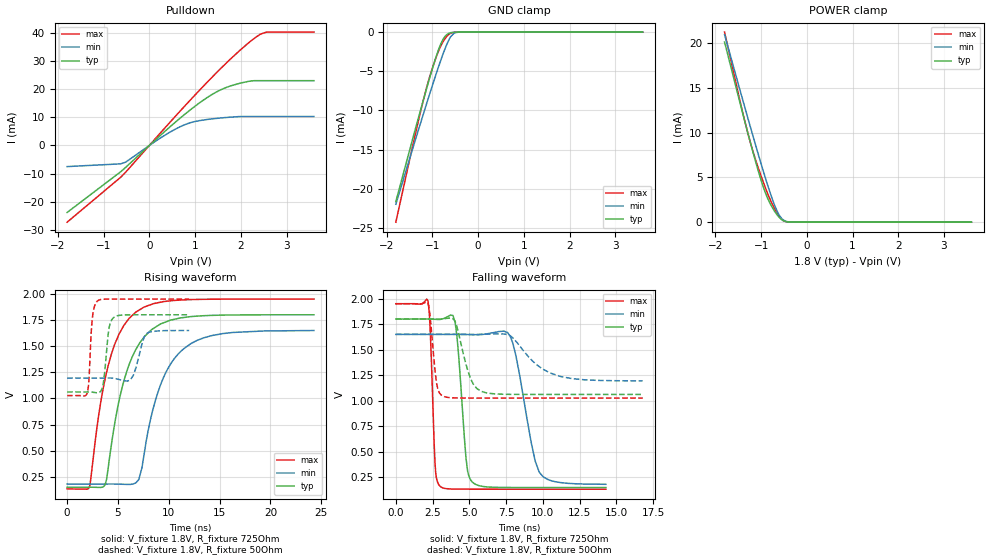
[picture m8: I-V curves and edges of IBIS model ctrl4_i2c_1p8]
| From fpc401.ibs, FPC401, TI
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|   ctrl4_i2c_1p8 Model
[Model]   ctrl4_i2c_1p8
Model_type   I/O_open_drain
Polarity   Non-Inverting
Vinl = 0.8
Vinh = 2
Vmeas = 0.9
Vref = 1.8
Cref = 50pF
Rref = 725
|   typ   min   max
|   (nom PVT)   (fast PVT)   (slow PVT)
C_comp   1.301e-14   1.196e-14   2.100e-14
| Where nom  PVT is Nominal Process, 1.8V, 27C
|   Fast PVT is Strong Process,  1.95V, -40C
|   Slow PVT is Weak Process,   1.65V, 125C
[Voltage Range]   1.8   1.65   1.95
|Junction Temperature
[Temperature Range]   27   125   -40
[Pullup Reference]   1.8   1.65   1.95
[Pulldown Reference]   0   0   0
[Power Clamp Reference]   1.8   1.65   1.95
[GND Clamp Reference]   0   0   0
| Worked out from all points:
|   slope of the pulldown table from 0 to 0.27 V, typ, clamps not added: 67.3 ohm
|   GND clamp passes 1 mA (typ) near -0.77 V on its own axis
|   POWER clamp passes 1 mA (typ) near -0.68 V on its own axis
|   falling waveform, V_fixture 1.8V, R_fixture 725Ohm: 20-80 % time 494ps typ, 1.1ns min, 265ps max; typ from 1.8 V to 0.152 V
|   rising waveform, V_fixture 1.8V, R_fixture 725Ohm: 20-80 % time 2.53ns typ, 2.78ns min, 2.33ns max; typ from 0.152 V to 1.8 V
|   falling waveform, V_fixture 1.8V, R_fixture 50Ohm: 20-80 % time 829ps typ, 2.01ns min, 364ps max; typ from 1.8 V to 1.06 V
|   rising waveform, V_fixture 1.8V, R_fixture 50Ohm: 20-80 % time 452ps typ, 746ps min, 317ps max; typ from 1.06 V to 1.8 V
[Pulldown]
|   Voltage   I(typ)   I(min)   I(max)
-1.8V     -23.87mA   -7.52mA    -27.33mA
-628mV    -9.35mA    -6.539mA   -11.32mA
-519.6mV  -7.811mA   -5.942mA   -9.523mA
251mV     3.762mA    2.768mA    4.649mA
682.2mV   9.87mA     6.746mA    12.43mA
1.012V    14.15mA    8.585mA    18.22mA
1.44V     18.83mA    9.603mA    25.46mA
1.649V    20.46mA    9.924mA    28.84mA
1.975V    22.16mA    10.31mA    33.83mA
2.434V    23.08mA    10.31mA    39.7mA
2.582V    23.08mA    10.31mA    40.39mA
3.6V      23.08mA    10.31mA    40.39mA
[GND Clamp]
|   Voltage   I(typ)   I(min)   I(max)
-1.8V     -21.65mA   -21.99mA   -24.29mA
-1.361V   -12.13mA   -13.55mA   -12.72mA
-1.207V   -8.874mA   -10.64mA   -8.916mA
-1.116V   -6.977mA   -8.932mA   -6.847mA
-973.2mV  -4.156mA   -6.328mA   -4.122mA
-889.2mV  -2.638mA   -4.838mA   -2.767mA
-823mV    -1.605mA   -3.705mA   -1.854mA
-725.4mV  -558.4uA   -2.145mA   -848.4uA
-630mV    -129.8uA   -881.8uA   -245.6uA
-522.9mV  -14.8uA    -128uA     -25.67uA
-437.1mV  -1.853uA   -14.05uA   -2.407uA
3.6V      0A         0A         0A
[POWER Clamp]
|   Voltage   I(typ)   I(min)   I(max)
-1.8V     20.14mA    20.97mA    21.24mA
-1.429V   12.69mA    14.15mA    12.83mA
-1.279V   9.754mA    11.44mA    9.727mA
-1.175V   7.762mA    9.566mA    7.842mA
-994.7mV  4.588mA    6.421mA    5.073mA
-849.6mV  2.58mA     4.012mA    3.098mA
-721.8mV  1.347mA    2.106mA    1.666mA
-637.2mV  733.1uA    1.09mA     899.8uA
-511.3mV  157.8uA    235.4uA    165.6uA
-404.1mV  16.52uA    35.43uA    12.03uA
-180mV    17.96nA    194.5nA    0A
3.6V      0A         0A         0A
[Ramp]
R_load = 725
|   typ   min   max
dV/dt_r   0.98887/2.53164e-09   0.880517/2.77844e-09   1.08855/2.33474e-09
dV/dt_f   0.988883/4.94199e-10   0.880513/1.10091e-09   1.08854/2.64772e-10
[Falling Waveform]
V_fixture = 1.8V
V_fixture_min = 1.65V
V_fixture_max = 1.95V
R_fixture = 725Ohm
|   Time   V(typ)   V(min)   V(max)
0s        1.8V       1.65V      1.95V
2.194ns   1.8V       1.65V      1.974V
2.665ns   1.798V     1.65V      389.5mV
3.022ns   1.797V     1.65V      163mV
4.038ns   1.764V     1.65V      136.4mV
4.772ns   439.8mV    1.649V     135.9mV
5.204ns   205.2mV    1.648V     135.8mV
7.78ns    152.1mV    1.633V     135.7mV
10.01ns   151.9mV    258.8mV    135.7mV
14.29ns   151.9mV    183.2mV    135.8mV
[Rising Waveform]
V_fixture = 1.8V
V_fixture_min = 1.65V
V_fixture_max = 1.95V
R_fixture = 725Ohm
|   Time   V(typ)   V(min)   V(max)
0s        151.8mV    182.5mV    135.7mV
2.194ns   152mV      182.5mV    153.1mV
3.73ns    173.9mV    182.5mV    1.183V
5.204ns   1.021V     180.9mV    1.632V
6.756ns   1.467V     194.1mV    1.825V
7.365ns   1.56V      338.7mV    1.861V
9.197ns   1.712V     1.132V     1.92V
11.49ns   1.774V     1.476V     1.943V
15.29ns   1.797V     1.62V      1.949V
24.28ns   1.8V       1.649V     1.95V
[Falling Waveform]
V_fixture = 1.8V
V_fixture_min = 1.65V
V_fixture_max = 1.95V
R_fixture = 50Ohm
|   Time   V(typ)   V(min)   V(max)
0s        1.8V       1.65V      1.95V
2.182ns   1.8V       1.65V      1.956V
2.781ns   1.799V     1.65V      1.163V
3.283ns   1.803V     1.65V      1.042V
4.043ns   1.774V     1.65V      1.029V
5.078ns   1.22V      1.65V      1.027V
5.83ns    1.092V     1.65V      1.027V
7.793ns   1.063V     1.636V     1.027V
11.23ns   1.062V     1.237V     1.027V
16.79ns   1.062V     1.195V     1.027V
[Rising Waveform]
V_fixture = 1.8V
V_fixture_min = 1.65V
V_fixture_max = 1.95V
R_fixture = 50Ohm
|   Time   V(typ)   V(min)   V(max)
0s        1.062V     1.195V     1.027V
1.959ns   1.063V     1.195V     1.047V
2.469ns   1.061V     1.195V     1.756V
2.97ns    1.054V     1.195V     1.93V
3.561ns   1.144V     1.195V     1.948V
4.141ns   1.681V     1.196V     1.95V
4.609ns   1.775V     1.193V     1.95V
6.218ns   1.799V     1.177V     1.95V
7.793ns   1.8V       1.619V     1.95V
12.01ns   1.8V       1.65V      1.95V
